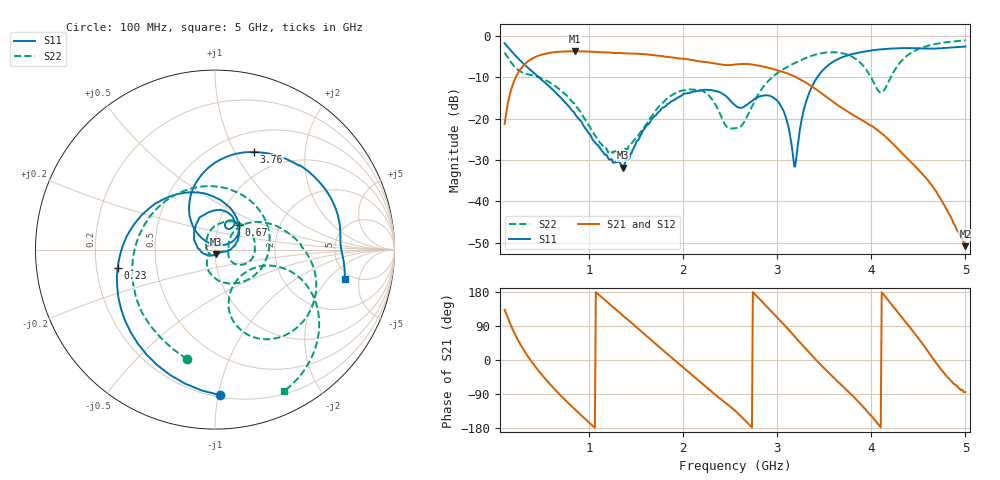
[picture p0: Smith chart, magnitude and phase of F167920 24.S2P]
!  2-Port S-parameters saved by WinCal
! VAR MeasName=S-Parameters (CALIBRATED_DATA) read from VNA (N5242A)
! VAR MeasDate=2016-11-22 9:56:21
! VAR NAME=F167920 24
! VAR FILENAME=F167920 24.S2P
! VAR DATE=2016-11-22 9:56:21
! VAR PHYS_PORTS=1,2
# Hz S DB R 50
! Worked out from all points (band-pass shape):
!   491 points, 100 MHz to 5 GHz, reference 50 ohm
!   highest |S21| = -3.72 dB at 850 MHz (marker M1); lowest = -50.8 dB at 5 GHz (marker M2)
!   |S21| within 3 dB of the highest: 321.1 MHz to 2.342 GHz (2.021 GHz wide, 152 % of centre)
!   lowest |S11| = -31.8 dB at 1.36 GHz (marker M3), VSWR 1.05, Z = 50.3 - j2.56 ohm
!   |S11| at or under -10 dB: 464.4 MHz to 3.426 GHz (2.961 GHz wide, 152 % of centre)
!   |S22| runs from -28.8 to -1.1 dB; largest |S21 - S12| = 0.00084
!   S11 on the Smith chart (normalised r, x): 100 MHz: 0.21, -1.02; 230 MHz: 0.29, -0.09; 670 MHz: 1.24, +0.36; 3.76 GHz: 0.72, +1.20; 5 GHz: 4.33, -3.15
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1e8  -1.81 -87.9  -21.33 132.3  -21.34 132.5  -4.02 -104.4
1.6e8  -3.39 -129.5  -13.79 95.3  -13.79 95.3  -6.13 -157.6
2.3e8  -5.15 -169.2  -9.50 58.5  -9.49 58.5  -8.00 145.6
4.3e8  -9.33 110.8  -5.10 -18.5  -5.09 -18.6  -9.78 29.9
6.7e8  -14.35 46.7  -3.88 -87.1  -3.88 -87.1  -12.68 -51.9
8.5e8  -18.96 11.2  -3.72 -131.2  -3.72 -131.2  -16.79 -97.0
9.2e8  -20.80 1.6  -3.75 -147.1  -3.75 -147.1  -18.75 -111.7
1.13e9  -27.59 -16.7  -3.98 166.0  -3.98 166.0  -26.17 -133.1
1.36e9  -31.82 -82.1  -4.21 116.7  -4.20 116.7  -28.00 -163.2
1.74e9  -18.36 157.8  -4.83 35.1  -4.83 35.0  -17.14 85.6
2.17e9  -13.25 91.4  -6.17 -55.9  -6.18 -56.0  -13.12 -4.3
2.55e9  -16.75 53.6  -6.93 -133.6  -6.94 -133.6  -22.33 3.5
2.75e9  -15.40 67.4  -7.00 176.6  -7.00 176.6  -16.09 44.0
2.99e9  -15.50 38.0  -8.27 114.6  -8.27 114.6  -9.20 24.0
3.19e9  -31.61 92.1  -9.86 60.9  -9.86 60.8  -6.53 4.7
3.37e9  -12.17 125.5  -12.27 11.1  -12.27 11.0  -4.79 -13.9
3.76e9  -4.64 68.2  -18.49 -84.6  -18.53 -84.6  -4.68 -58.9
3.99e9  -3.59 45.1  -21.64 -145.2  -21.67 -145.1  -9.85 -76.6
4.1e9  -3.28 36.6  -23.40 -177.9  -23.46 -177.6  -13.74 -47.7
4.19e9  -3.12 29.7  -25.24 154.3  -25.27 154.4  -10.77 -18.2
4.49e9  -3.01 9.7  -32.08 60.8  -32.16 60.7  -3.31 -32.3
5e9  -2.61 -12.8  -50.83 -85.0  -51.01 -86.9  -1.13 -64.1
